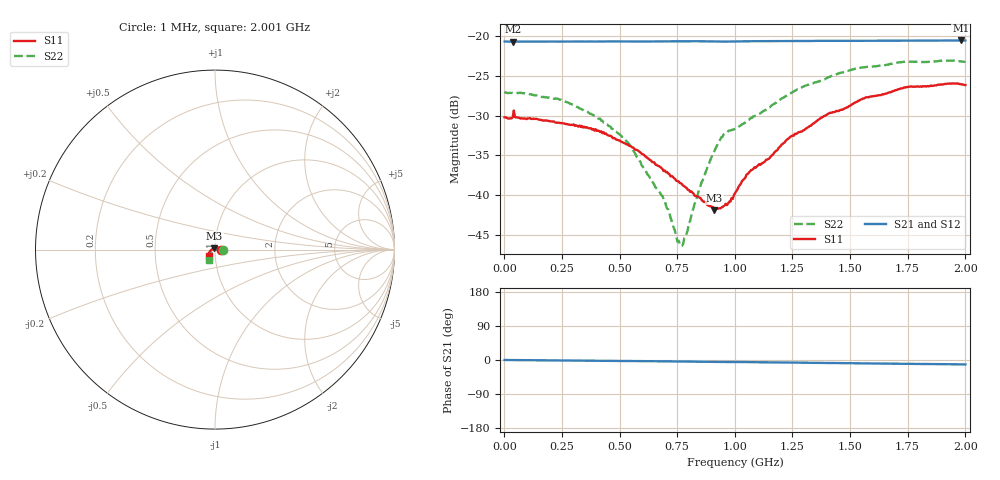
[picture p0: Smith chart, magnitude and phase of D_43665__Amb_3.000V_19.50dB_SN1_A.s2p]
! device id: 43665_
! dir: \\malibu\benchdata\1_engineers\tn_data\43665_75ohm\new\sparar\43665_\amb\3p000v\19p50db
! Serial: 1
! Insertion: A
! Temp: Amb
! VDD: 3.000V
! Attenuation Step: 19.50dB
! IDD: 1.452409e+00mA
! FILE NAME
! DATE 03-27-2009 08:38:08
! CORRECTED  DATA
#  Hz  S  RI  R  75
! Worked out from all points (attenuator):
!   401 points, 1 MHz to 2.001 GHz, reference 75 ohm
!   highest |S21| = -20.53 dB at 1.981 GHz (marker M1); lowest = -20.7 dB at 36 MHz (marker M2)
!   lowest |S11| = -41.9 dB at 911 MHz (marker M3), VSWR 1.02, Z = 74.5 + j1.09 ohm
!   |S11| at or under -10 dB: start of sweep to end of sweep
!   |S22| runs from -46.5 to -23.1 dB; largest |S21 - S12| = 0.00076
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1000000  0.0309 -0.000202  0.0926 -0.000124  0.0927 -1.85e-05  0.0448 -0.000472
3.6e7  0.0309 0.00114  0.0925 -0.000263  0.0925 -0.000275  0.044 0.000636
2.36e8  0.0279 0.00618  0.0926 -0.00176  0.0926 -0.0018  0.0397 0.00576
3.36e8  0.0261 0.00806  0.0926 -0.00257  0.0927 -0.00268  0.0339 0.00723
5.26e8  0.0181 0.0108  0.0927 -0.00421  0.0927 -0.00438  0.0217 0.00462
6.71e8  0.0105 0.011  0.0926 -0.00538  0.0927 -0.00554  0.0105 0.000214
7.06e8  0.00885 0.0108  0.0927 -0.00574  0.0927 -0.00589  0.00814 -0.000958
7.56e8  0.00617 0.0105  0.0928 -0.00624  0.0928 -0.00643  0.00399 -0.00326
7.71e8  0.00542 0.0104  0.0927 -0.00643  0.0928 -0.00658  0.0026 -0.00401
7.86e8  0.00464 0.0102  0.0928 -0.00661  0.0927 -0.00678  0.00134 -0.00526
8.51e8  0.000853 0.00952  0.0927 -0.00737  0.0927 -0.00754  -0.00345 -0.0109
9.11e8  -0.00323 0.00734  0.0924 -0.00804  0.0925 -0.00821  -0.00907 -0.0165
9.51e8  -0.00551 0.00646  0.0922 -0.00822  0.0922 -0.00835  -0.0155 -0.0184
1.001e9  -0.00844 0.00582  0.0924 -0.00833  0.0924 -0.00854  -0.0194 -0.0174
1.076e9  -0.0141 0.00304  0.0927 -0.00933  0.0927 -0.00951  -0.0212 -0.0222
1.236e9  -0.0226 -0.00328  0.0926 -0.0109  0.0927 -0.0112  -0.0266 -0.034
1.336e9  -0.0267 -0.00803  0.0927 -0.0119  0.0928 -0.0122  -0.03 -0.0407
1.556e9  -0.0348 -0.0208  0.0925 -0.0145  0.0927 -0.0148  -0.0339 -0.0538
1.671e9  -0.036 -0.0259  0.0925 -0.0157  0.0926 -0.0161  -0.0349 -0.0567
1.756e9  -0.0363 -0.0314  0.0924 -0.0166  0.0926 -0.0171  -0.0342 -0.0602
1.981e9  -0.0327 -0.0377  0.0922 -0.0188  0.0922 -0.0195  -0.0336 -0.0609
2.001e9  -0.0318 -0.0376  0.0921 -0.019  0.092 -0.0196  -0.0335 -0.0601
